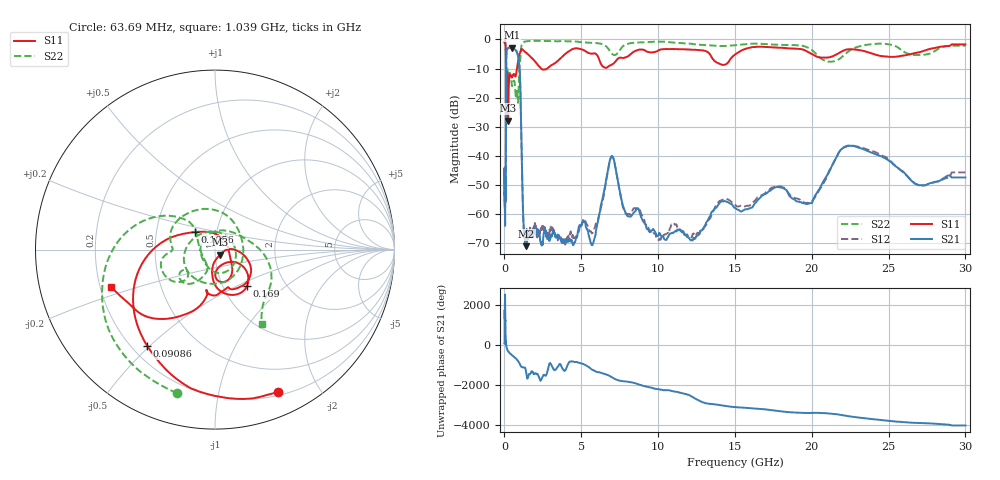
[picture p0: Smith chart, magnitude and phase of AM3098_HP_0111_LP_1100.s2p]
! Date/Time: Thu, Feb 28, 2019 8:39 AM
! Network Analyzer: Agilent Technologies E8364B Rev: A.07.50.67
! Sweep from 0.010 to 30.000 GHz, 1601 Points, Sweep Type: LOG
! Power Supply: 5.023 V, 0.002 A
# Hz S DB R 50
!freq MagS11 AngS11 MagS21 AngS21 MagS12 AngS12 MagS22 AngS22
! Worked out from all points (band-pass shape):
!   1601 points, 10 MHz to 30 GHz, reference 50 ohm
!   highest |S21| = -2.81 dB at 478.5 MHz (marker M1); lowest = -71.0 dB at 1.424 GHz (marker M2)
!   |S21| within 3 dB of the highest: 121.9 MHz to 889.1 MHz (767.2 MHz wide, 152 % of centre)
!   lowest |S11| = -27.9 dB at 238.7 MHz (marker M3), VSWR 1.08, Z = 52.8 - j3.04 ohm
!   |S11| at or under -10 dB: 102.2 MHz to 811.6 MHz (709.4 MHz wide, 155 % of centre); 2.374 GHz to 2.779 GHz (404.1 MHz wide, 15.7 % of centre)
!   |S22| runs from -22.2 to -0.5 dB; largest |S21 - S12| = 0.011
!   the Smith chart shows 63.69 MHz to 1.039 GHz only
!   S11 on the Smith chart (normalised r, x): 63.69 MHz: 0.24, -1.51; 90.86 MHz: 0.26, -0.49; 105.6 MHz: 0.78, +0.16; 169 MHz: 1.29, -0.57; 1.039 GHz: 0.25, -0.16
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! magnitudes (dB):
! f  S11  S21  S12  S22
! 10 MHz  -0.4  -44.4  -43.8  -0.6
! 38.04 MHz  -0.5  -61.1  -61.9  -0.9
! 63.69 MHz  -1.3  -54.3  -52.3  -1.6
! 90.86 MHz  -3.7  -45.1  -44.5  -4.0
! 105.6 MHz  -16.5  -14.2  -14.2  -20.6
! 144.7 MHz  -19.9  -4.0  -3.9  -14.1
! 169 MHz  -11.4  -3.5  -3.5  -10.6
! 238.7 MHz  -27.9  -2.9  -2.9  -12.2
! 478.5 MHz  -13.1  -2.8  -2.8  -15.7
! 550.5 MHz  -12.3  -3.1  -3.0  -14.9
! 885.5 MHz  -7.7  -5.7  -5.7  -21.7
! 1.039 GHz  -4.2  -17.8  -17.8  -6.2
! 1.232 GHz  -3.7  -61.9  -63.5  -1.0
! 1.424 GHz  -4.6  -71.0  -67.1  -0.6
! 2.084 GHz  -8.2  -67.2  -66.1  -0.5
! 5.725 GHz  -4.9  -70.7  -66.5  -1.2
! 6.994 GHz  -8.7  -40.0  -40.2  -4.9
! 7.926 GHz  -6.1  -60.1  -59.7  -1.7
! 12.19 GHz  -3.5  -68.9  -68.0  -1.5
! 19.8 GHz  -4.4  -56.4  -56.3  -3.0
! 22.56 GHz  -3.4  -36.5  -36.5  -3.5
! 30 GHz  -1.7  -47.4  -45.7  -2.2
